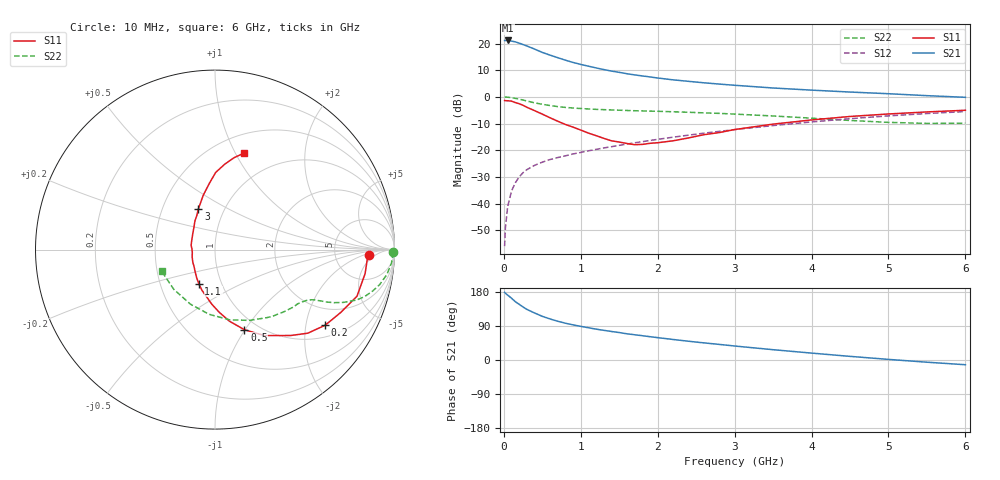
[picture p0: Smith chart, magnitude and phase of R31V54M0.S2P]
! SIEMENS Small Signal Semiconductors
! BFR181
! Si NPN RF Bipolar Junction Transistor in SOT23
! VCE = 1.5 V  IC = 4 mA
! Common Emitter S-Parameters:  May  1996
# GHz  S  MA  R  50
!  f  S11  S21  S12  S22
! GHz  MAG  ANG  MAG  ANG  MAG  ANG  MAG  ANG
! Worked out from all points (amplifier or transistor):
!   36 points, 10 MHz to 6 GHz, reference 50 ohm
!   highest |S21| = 21.1 dB at 50 MHz (marker M1)
!   |S21| within 3 dB of that: start of sweep to 379.6 MHz
!   unconditionally stable (mu >= 1): 1.158 GHz to 3.083 GHz
!   at 250 MHz: K = 0.37, MSG = 24.0 dB, |S12| = -28.4 dB
!   at 1.4 GHz: K = 1.05, MAG = 12.8 dB, |S12| = -18.7 dB
!   at 6 GHz: K = 0.86, MSG = 2.7 dB, |S12| = -5.5 dB
!   S11 on the Smith chart (normalised r, x): 10 MHz: 12, -3; 200 MHz: 1.36, -2.58; 500 MHz: 0.86, -0.99; 1.1 GHz: 0.78, -0.31; 3 GHz: 0.76, +0.36; 6 GHz: 0.69, +1.09
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0.01  0.8569 -2.0  11.38 178.4  0.0016 96.9  0.9932 -0.9
0.02  0.8496 -4.0  11.39 176.2  0.0035 80.7  0.9905 -1.8
0.05  0.8469 -9.1  11.41 171.2  0.0089 85.3  0.9864 -4.3
0.1  0.8327 -18.2  11.09 163.0  0.0173 79.8  0.9681 -8.2
0.15  0.7824 -26.7  10.74 153.8  0.0247 75.0  0.938 -12.0
0.2  0.7444 -34.5  10.15 146.9  0.0318 72.2  0.9061 -14.9
0.25  0.6959 -42.0  9.557 139.9  0.0381 68.5  0.8731 -17.5
0.3  0.6382 -48.6  8.987 133.5  0.0434 66.9  0.8373 -19.6
0.4  0.5525 -60.1  7.857 124.0  0.0523 62.9  0.7747 -22.3
0.5  0.4757 -69.8  6.806 115.2  0.0599 61.2  0.727 -24.0
0.6  0.407 -78.6  6.063 108.4  0.0671 60.3  0.689 -25.1
0.7  0.3504 -86.1  5.431 102.3  0.0731 60.0  0.6585 -25.8
0.8  0.3045 -93.4  4.876 97.1  0.0787 59.9  0.6361 -26.4
0.9  0.2714 -99.2  4.417 92.7  0.0854 60.1  0.6187 -26.9
1.1  0.2098 -115.6  3.761 85.1  0.0978 60.5  0.5941 -28.2
1.6  0.1341 -161.7  2.717 69.2  0.1307 61.5  0.5569 -32.3
2.2  0.1505 145.9  2.087 54.2  0.1759 60.8  0.5264 -39.6
3  0.2448 112.2  1.651 36.9  0.2438 56.6  0.4765 -52.7
3.5  0.3091 102.3  1.468 27.2  0.2905 52.9  0.4392 -63.9
4.5  0.43 89.5  1.233 9.6  0.3906 42.6  0.362 -95.2
5.5  0.5229 78.3  1.055 -5.8  0.4884 29.7  0.319 -136.0
6  0.5619 73.2  0.982 -12.5  0.5313 22.5  0.3209 -157.9
